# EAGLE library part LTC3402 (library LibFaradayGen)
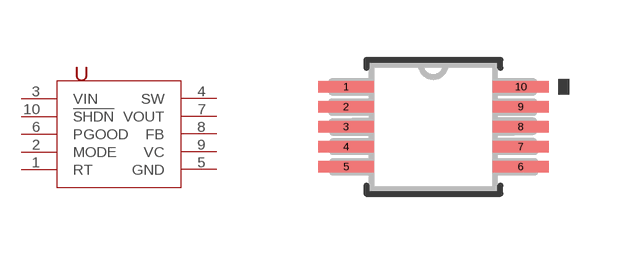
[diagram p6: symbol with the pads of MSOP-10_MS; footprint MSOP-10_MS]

Designator prefix U

## LTC3402  [MSOP-10_MS]
1  RT  out
2  MODE  out
3  VIN  out
4  SW  out
5  GND  out
6  PGOOD  out
7  VOUT  out
8  FB  out
9  VC  out
10  !SHDN!  out

## Footprint MSOP-10_MS (pad centres in mm)
smd 1.397 x 0.279: 1 -2.184,1.001; 2 -2.184,0.5; 3 -2.184,0; 4 -2.184,-0.5; 5 -2.184,-1.001; 6 2.184,-1.001; 7 2.184,-0.5; 8 2.184,0; 9 2.184,0.5; 10 2.184,1.001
